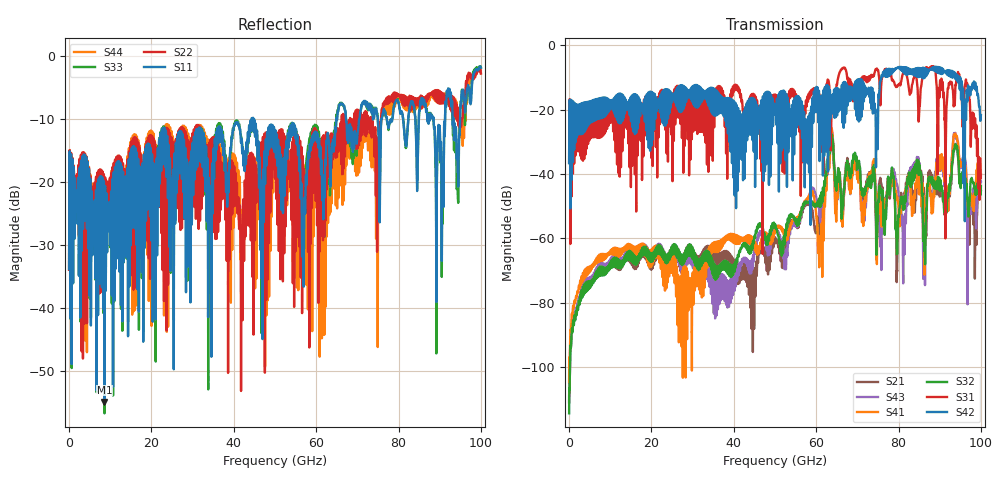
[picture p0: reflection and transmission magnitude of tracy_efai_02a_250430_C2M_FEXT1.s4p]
!! PART DESCRIPTION: TE 224G+ VSR Channel- Chip to module, IO connector to CPC(Co-packaged connector) through over the board cable
!! CHANNEL DESCRIPTION: Module trace -> Mated IO 224G+ Connector -> Internal Cable Termination -> 30AWG 300mm Cable -> Cable
!!  termination + CPC connector(No footprint or package included)
!! MODEL REVISION:  Rev 3, Created on April 29, 2025
!! MODEL STATUS: Development
!! MODEL GEOMETRY: FEXT1
!! MODEL FREQUENCY RANGE: 0 GHz to 100 GHz in 10.00 MHz frequency steps
!! PORT DEFINITIONS:
!! Port  1  ----->  Module Side  -->  Host Side  <-----  Port  2
!! Port  3  ----->  Module Side  -->  Host Side  <-----  Port  4
# HZ S MA R 45.000000
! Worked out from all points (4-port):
!   10000 points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, 10 MHz to 100 GHz, reference 45 ohm
!   strongest paths, dB at 10 MHz, 25.01 GHz, 50.01 GHz, 75.01 GHz, 100 GHz:
!     S42: -36.7, -17.7, -20.3, -22.6, -21.7
!     S31: -36.5, -17.8, -16.0, -7.7, -40.6
!     S32: -114.4, -65.2, -55.8, -49.1, -43.8
!     S41: -104.7, -68.1, -58.0, -52.5, -40.0
!     S43: -111.2, -65.7, -57.4, -49.6, -42.3
!     S21: -110.7, -66.5, -60.1, -48.2, -45.0
!   lowest |S11| = -54.9 dB at 8.6 GHz (marker M1), VSWR 1.00, Z = 44.9 + j0.15 ohm
!   |S11| at or under -10 dB: start of sweep to 44.32 GHz; 44.72 GHz to 64.9 GHz (20.18 GHz wide, 36.8 % of centre); 67.23 GHz to 70.41 GHz (3.185 GHz wide, 4.63 % of centre)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
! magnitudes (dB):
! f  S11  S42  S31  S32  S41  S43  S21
! 10 MHz  -33.8  -36.7  -36.5  -114.4  -104.7  -111.2  -110.7
! 8.6 GHz  -54.9  -22.2  -27.5  -70.3  -65.4  -68.7  -69.5
! 44.78 GHz  -11.1  -20.5  -15.6  -61.4  -62.5  -66.4  -70.6
! 61.02 GHz  -14.4  -18.2  -17.0  -46.7  -60.3  -50.8  -50.6
! 63.77 GHz  -14.4  -18.1  -18.5  -27.6  -25.8  -26.1  -27.3
! 88.17 GHz  -9.4  -7.6  -7.5  -41.0  -51.9  -48.6  -40.5
! 100 GHz  -1.8  -21.7  -40.6  -43.8  -40.0  -42.3  -45.0
